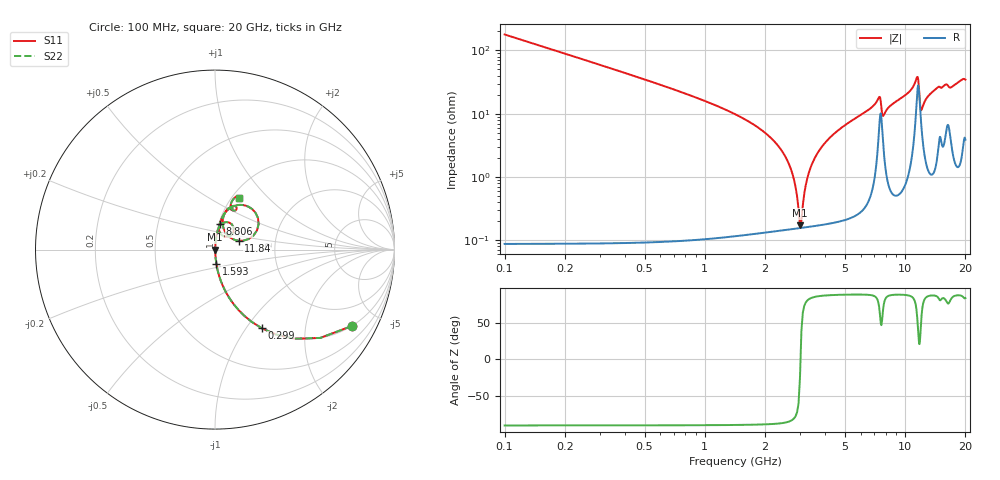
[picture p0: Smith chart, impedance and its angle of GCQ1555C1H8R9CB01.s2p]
!Murata Part Number: GCQ1555C1H8R9CB01
!These Parameters are Measured in Series Mode Connection
!Data Generated on Jan 08, 2026
!  o--ll--o
!Port1  Port2
!  o------o
!Operation Temp=25[degC], DC Bias Voltage=0[V]
!Freq. Start=100[MHz] Stop=20[GHz] 401[Steps]
# Hz S RI R 50
!Freq.(Hz) S11(Real) S11(Imag) S21(Real) S21(Imag) S12(Real) S12(Imag) S22(Real) S22(Imag)
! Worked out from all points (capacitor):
!   401 points, 100 MHz to 20 GHz, reference 50 ohm
!   read as one part in series: C = 8.9 pF near 199.5 MHz
!   lowest |Z| = 171 mohm at 2.986 GHz (marker M1)
!   series resonance near 3.003 GHz, so ESL is about 320 pH
!   S11 on the Smith chart (normalised r, x): 100 MHz: 1.00, -3.57; 299 MHz: 1.00, -1.18; 1.593 GHz: 1.00, -0.16; 8.806 GHz: 1.01, +0.30; 11.84 GHz: 1.30, +0.13; 20 GHz: 1.08, +0.69
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1e8  0.7613 -0.4261  0.2387 0.4261  0.2387 0.4261  0.7613 -0.4261
2.99e8  0.2599 -0.4378  0.7401 0.4378  0.7401 0.4378  0.2599 -0.4378
6.4725e8  0.0657 -0.2459  0.9343 0.2459  0.9343 0.2459  0.0657 -0.2459
1.5925e9  0.00766 -0.08  0.9923 0.08  0.9923 0.08  0.00766 -0.08
2.53775e9  0.00186 -0.0202  0.9981 0.0202  0.9981 0.0202  0.00186 -0.0202
2.73675e9  0.00162 -0.0111  0.9984 0.0111  0.9984 0.0111  0.00162 -0.0111
2.9855e9  0.00156 -0.000707  0.9984 0.000707  0.9984 0.000707  0.00156 -0.000707
3.085e9  0.00159 0.00321  0.9984 -0.00321  0.9984 -0.00321  0.00159 0.00321
3.23425e9  0.00169 0.00888  0.9983 -0.00888  0.9983 -0.00888  0.00169 0.00888
3.43325e9  0.00191 0.0161  0.9981 -0.0161  0.9981 -0.0161  0.00191 0.0161
4.478e9  0.00438 0.0497  0.9956 -0.0497  0.9956 -0.0497  0.00438 0.0497
6.7665e9  0.0202 0.1207  0.9798 -0.1207  0.9798 -0.1207  0.0202 0.1207
7.41325e9  0.0785 0.1507  0.9215 -0.1507  0.9215 -0.1507  0.0785 0.1507
7.7615e9  0.0403 0.0791  0.9597 -0.0791  0.9597 -0.0791  0.0403 0.0791
8.80625e9  0.0263 0.1438  0.9737 -0.1438  0.9737 -0.1438  0.0263 0.1438
1.005e10  0.0445 0.1875  0.9555 -0.1875  0.9555 -0.1875  0.0445 0.1875
1.1443e10  0.2077 0.2253  0.7923 -0.2253  0.7923 -0.2253  0.2077 0.2253
1.1841e10  0.1316 0.0493  0.8684 -0.0493  0.8684 -0.0493  0.1316 0.0493
1.204e10  0.0699 0.0805  0.9301 -0.0805  0.9301 -0.0805  0.0699 0.0805
1.338325e10  0.0506 0.1942  0.9494 -0.1942  0.9494 -0.1942  0.0506 0.1942
1.67165e10  0.0996 0.2179  0.9004 -0.2179  0.9004 -0.2179  0.0996 0.2179
2e10  0.1321 0.2869  0.8679 -0.2869  0.8679 -0.2869  0.1321 0.2869
